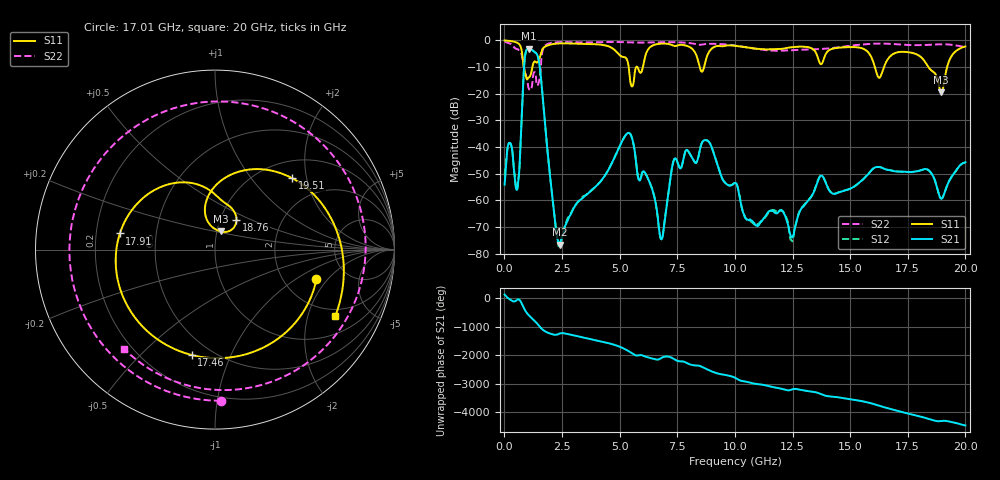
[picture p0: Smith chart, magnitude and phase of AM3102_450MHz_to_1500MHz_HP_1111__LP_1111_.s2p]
!Agilent Technologies,E8364B,MY43040894,A.07.50.67
!Agilent E8364B: A.07.50.67
!Date: Thursday, January 11, 2018 06:52:43
!Correction: S11(Full 2 Port(1,2))
!S21(Full 2 Port(1,2))
!S12(Full 2 Port(1,2))
!S22(Full 2 Port(1,2))
!S2P File: Measurements: S11, S21, S12, S22:
# Hz S  dB  R 50
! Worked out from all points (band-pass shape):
!   1601 points, 10 MHz to 20 GHz, reference 50 ohm
!   highest |S21| = -3.15 dB at 1.072 GHz (marker M1); lowest = -76.7 dB at 2.396 GHz (marker M2)
!   |S21| within 3 dB of the highest: 893 MHz to 1.454 GHz (560.7 MHz wide, 47.8 % of centre)
!   lowest |S11| = -19.5 dB at 18.95 GHz (marker M3), VSWR 1.24, Z = 52.1 + j10.7 ohm
!   |S11| at or under -10 dB: 842 MHz to 1.216 GHz (374.1 MHz wide, 36.4 % of centre); 16.07 GHz to 16.47 GHz (396 MHz wide, 2.43 % of centre); 18.39 GHz to 19.21 GHz (817.7 MHz wide, 4.35 % of centre)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
!   |S22| runs from -18.7 to -0.5 dB; largest |S21 - S12| = 0.0021
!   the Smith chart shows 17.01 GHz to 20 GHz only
!   S11 on the Smith chart (normalised r, x): 17.01 GHz: 3.01, -1.53; 17.46 GHz: 0.39, -0.72; 17.91 GHz: 0.30, +0.08; 18.76 GHz: 1.20, +0.41; 19.51 GHz: 1.36, +1.65; 20 GHz: 1.69, -3.02
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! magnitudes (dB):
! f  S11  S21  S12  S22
! 10 MHz  -0.1  -54.2  -50.7  -0.5
! 234.9 MHz  -0.3  -38.5  -38.5  -1.2
! 572.2 MHz  -1.0  -55.2  -55.1  -3.3
! 884.6 MHz  -11.8  -6.8  -6.8  -11.2
! 1.072 GHz  -13.9  -3.1  -3.2  -18.3
! 1.509 GHz  -7.1  -8.5  -8.5  -15.1
! 2.396 GHz  -1.2  -76.7  -76.7  -0.7
! 3.346 GHz  -1.4  -59.5  -59.0  -0.8
! 5.395 GHz  -10.1  -34.7  -34.7  -0.8
! 6.682 GHz  -1.4  -68.7  -68.8  -0.7
! 8.668 GHz  -9.9  -37.5  -37.5  -1.5
! 10.01 GHz  -2.1  -53.5  -53.4  -2.0
! 12.47 GHz  -2.6  -73.9  -75.2  -3.7
! 13.34 GHz  -3.1  -58.3  -58.2  -3.4
! 16.68 GHz  -6.6  -48.6  -48.6  -1.3
! 17.01 GHz  -4.6  -49.2  -49.2  -1.5
! 17.46 GHz  -4.4  -49.4  -49.4  -1.7
! 17.91 GHz  -5.4  -49.1  -49.1  -1.8
! 18.76 GHz  -13.9  -55.0  -55.0  -1.6
! 18.95 GHz  -19.5  -59.4  -59.3  -1.5
! 19.51 GHz  -4.6  -49.9  -49.9  -1.8
! 20 GHz  -2.3  -45.8  -45.9  -2.5
